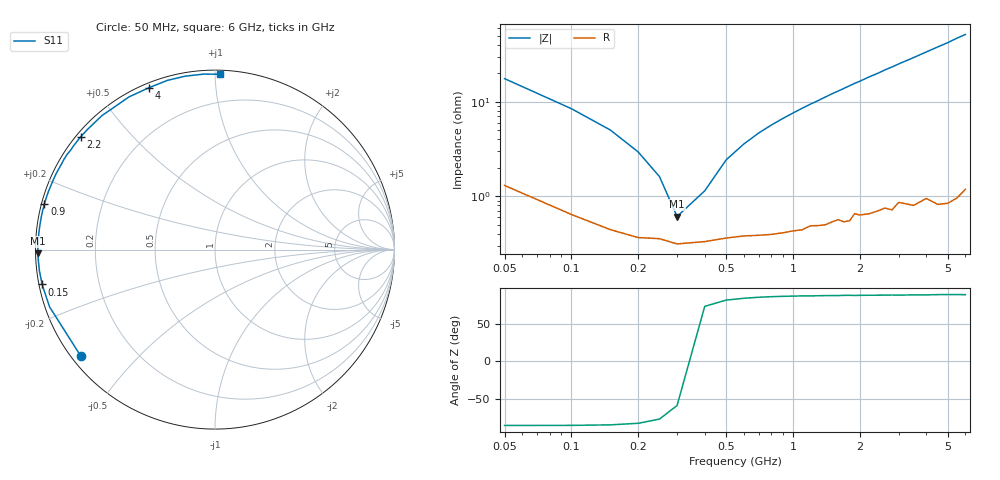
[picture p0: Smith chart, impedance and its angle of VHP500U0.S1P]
! Infineon Technologies  Discrete & RF Semiconductors
! BB 814
! Si Tuning Diode in SOT23
! VR = 0.5 V
! S-Parameters:  July  1999
# GHz  S  MA  R  50
!  f  S11
! GHz  MAG  ANG
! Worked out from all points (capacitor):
!   34 points, 50 MHz to 6 GHz, reference 50 ohm
!   read as one part to ground: C = 172 pF near 50 MHz
!   lowest |Z| = 610 mohm at 300 MHz (marker M1)
!   series resonance near 332.4 MHz, so ESL is about 1.3 nH
!   S11 on the Smith chart (normalised r, x): 50 MHz: 0.03, -0.35; 150 MHz: 0.01, -0.10; 900 MHz: 0.01, +0.13; 2.2 GHz: 0.01, +0.36; 4 GHz: 0.02, +0.67; 6 GHz: 0.02, +1.03
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0.05  0.9547 -141.5
0.1  0.9754 -160.9
0.15  0.9826 -168.6
0.2  0.9855 -173.3
0.25  0.9859 -176.4
0.3  0.9876 -178.8
0.4  0.9868 177.5
0.5  0.9857 174.5
0.7  0.9848 169.4
0.8  0.9845 167.1
0.9  0.984 164.9
1.2  0.9814 158.7
1.5  0.98 152.8
1.6  0.979 151.0
1.8  0.98 147.2
1.9  0.9765 145.3
2  0.9774 143.7
2.2  0.9772 140.0
2.4  0.9762 136.8
2.6  0.975 133.2
2.8  0.9767 130.1
3  0.9728 126.8
3.5  0.9764 119.4
4  0.9742 112.3
4.5  0.9794 105.7
5  0.9805 99.8
5.5  0.9798 93.6
6  0.9772 88.5
